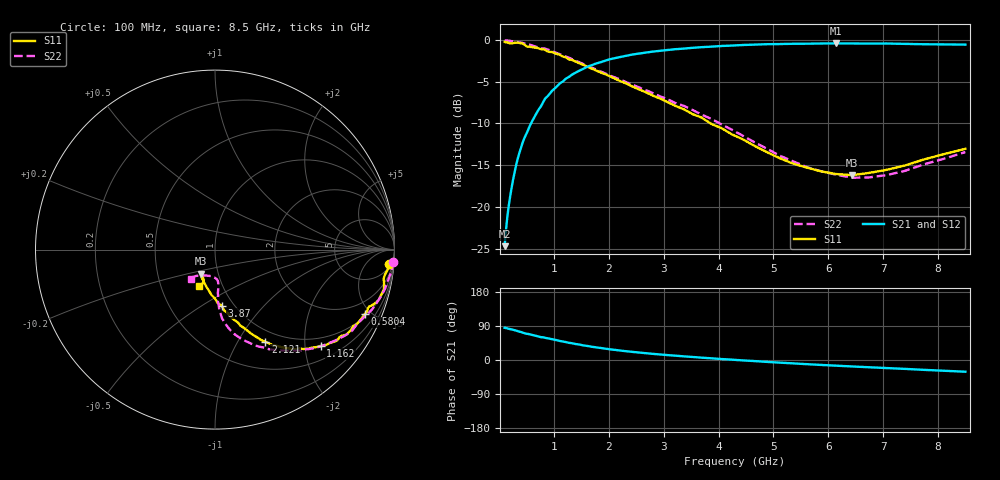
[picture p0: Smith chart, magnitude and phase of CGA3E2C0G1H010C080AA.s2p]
! S-parameter Generated by TDK Corporation
! Copyright(C) 2015 TDK Corporation.
! All Rights Reserved.
! TDK P/N: CGA3E2C0G1H010C080AA (Multilayer Ceramic Chip Capacitors)
! Property: C=1pF
! Size(LxWxT): 1.6x0.8x0.8mm, 0.063x0.031x0.031inches
! Model Type: s2p (Touchstone File Format Version 1.0)
! Frequency: DC=Yes Start=100MHz Stop=8500MHz 98points Log-sweep
! Note:
! Model Generated on Jun. 23, 2015
! Hash(MD5):
! Port Assignments:
!  1 ---| |--- 2
! Applicable Conditions:
!  Temperature = 25 degC
!  DC Bias Voltage = 0 V
!  Small Signal Operation
! Terms and conditions regarding TDK Simulation Models
! (1)This simulation model is being provided solely for informational purposes. Please refer to the specifications of the products in terms of detailed characteristics of such products.
! (2)In no event shall TDK Corporation of any of its subsidiaries be liable for any loss or damage arising, directly or indirectly,
!  From any information contained in this simulation model, including, but not limited to loss or damages arising from any inaccuracies, omissions or errors in connection with such information.
! (3)Any and all copyrights on this simulation model are owned by TDK Corporation.
!  Duplication or redistribution of this simulation model without prior written permission from TDK Corporation is prohibited.
! (4)This simulation model is subject to any modification or change without any prior notice.
! (5)Neither TDK Corporation nor any of its subsidiaries shall make any warranty, express or implied,
!  Including but not limited to the correctness, implied warranties of merchantability and fitness for a particular purpose with respect to this simulation models.
! (6)The use of this simulation model shall be deemed to have consented to the terms and conditions hereof.
# MHz S MA R 50
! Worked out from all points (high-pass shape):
!   97 points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, 100 MHz to 8.5 GHz, reference 50 ohm
!   highest |S21| = -0.40 dB at 6.148 GHz (marker M1); lowest = -24.7 dB at 100 MHz (marker M2)
!   |S21| within 3 dB of the highest: 1.549 GHz to end of sweep
!   lowest |S11| = -16.2 dB at 6.439 GHz (marker M3), VSWR 1.37, Z = 41.5 - j11.4 ohm
!   |S11| at or under -10 dB: 3.856 GHz to end of sweep
!   |S22| runs from -16.5 to 0.0 dB; largest |S21 - S12| = 0.0044
!   S11 on the Smith chart (normalised r, x): 100 MHz: 7, -23; 580.4 MHz: 1.11, -4.58; 1.162 GHz: 0.80, -2.34; 2.121 GHz: 0.84, -1.31; 3.87 GHz: 0.88, -0.61; 8.5 GHz: 0.77, -0.33
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100  0.9752 -4.6  0.05818 85.1  0.05824 85.1  0.9937 -3.9
138.2569  0.9712 -6.1  0.08023 84.0  0.08007 84.1  0.9916 -5.2
174.2518  0.9605 -7.8  0.1007 82.4  0.1006 82.5  0.9917 -6.6
289.9056  0.9625 -11.9  0.1658 78.4  0.1657 78.4  0.9776 -10.9
419.7991  0.9547 -17.0  0.238 72.8  0.2382 72.8  0.9617 -15.7
505.1658  0.9154 -20.3  0.2777 69.2  0.2781 69.2  0.9462 -18.6
580.4012  0.9082 -23.3  0.3159 66.9  0.3156 66.9  0.9335 -21.3
766.1556  0.88 -28.9  0.4024 60.2  0.4023 60.2  0.8937 -27.4
840.4526  0.8724 -32.9  0.4464 58.7  0.4458 58.6  0.8874 -30.6
1161.984  0.7959 -42.4  0.5645 48.8  0.5654 48.7  0.8105 -40.9
1533.871  0.7096 -51.5  0.6723 38.5  0.6729 38.6  0.7183 -51.6
2120.682  0.5848 -61.4  0.7804 26.5  0.7803 26.5  0.5952 -65.4
2551.925  0.5057 -67.0  0.8301 19.7  0.8301 19.8  0.5198 -73.3
2931.989  0.4468 -71.5  0.862 14.6  0.8623 14.6  0.4603 -78.9
3870.357  0.3139 -83.3  0.913 4.4  0.912 4.6  0.3369 -85.9
4446.777  0.2538 -94.4  0.934 -1.1  0.9326 -0.9  0.2666 -86.1
5351.035  0.1821 -112.1  0.9498 -8.9  0.9501 -8.9  0.1882 -84.3
5869.945  0.1634 -119.0  0.9535 -13.0  0.9509 -12.9  0.1635 -87.2
6147.976  0.1574 -119.7  0.9549 -15.0  0.9542 -14.9  0.156 -90.8
6439.175  0.155 -119.6  0.9539 -17.1  0.9513 -16.9  0.1496 -96.8
7398.175  0.1772 -110.8  0.9486 -23.5  0.9488 -23.6  0.1645 -119.4
8500  0.223 -113.5  0.9391 -30.9  0.9398 -30.8  0.2132 -128.8
